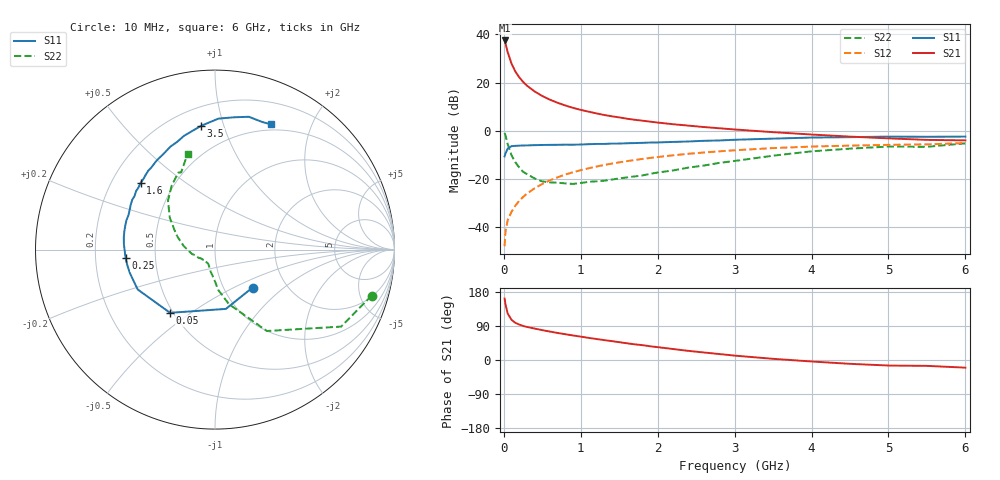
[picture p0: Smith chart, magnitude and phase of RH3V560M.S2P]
! SIEMENS Small Signal Semiconductors
! BFR106
! Si NPN RF Bipolar Junction Transistor in SOT23
! VCE = 3.5 V  IC = 60 mA
! Common Emitter S-Parameters:  August  1996
# GHz  S  MA  R  50
!  f  S11  S21  S12  S22
! GHz  MAG  ANG  MAG  ANG  MAG  ANG  MAG  ANG
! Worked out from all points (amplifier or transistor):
!   36 points, 10 MHz to 6 GHz, reference 50 ohm
!   highest |S21| = 37.5 dB at 10 MHz (marker M1)
!   |S21| within 3 dB of that: start of sweep to 35.55 MHz
!   unconditionally stable (mu >= 1): 220.8 MHz to 2.416 GHz
!   at 250 MHz: K = 1.02, MAG = 22.9 dB, |S12| = -27.4 dB
!   at 1.4 GHz: K = 1.06, MAG = 8.4 dB, |S12| = -13.5 dB
!   at 6 GHz: K = 0.99, MSG = 0.6 dB, |S12| = -5.0 dB
!   S11 on the Smith chart (normalised r, x): 10 MHz: 1.36, -0.63; 50 MHz: 0.48, -0.42; 250 MHz: 0.33, -0.04; 1.6 GHz: 0.32, +0.35; 3.5 GHz: 0.32, +0.84; 6 GHz: 0.43, +1.45
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0.01  0.2975 -45.3  75.12 162.1  0.0041 81.5  0.9091 -16.4
0.02  0.3359 -79.6  66.84 148.0  0.0079 69.0  0.8234 -31.4
0.05  0.4321 -125.4  43 122.6  0.0142 61.3  0.5378 -57.5
0.1  0.4846 -152.7  24.83 105.9  0.0212 63.7  0.3139 -75.6
0.15  0.4918 -164.4  17.03 98.0  0.0284 66.3  0.2245 -85.6
0.2  0.4962 -169.9  12.98 93.6  0.0356 69.0  0.1751 -90.3
0.25  0.5004 -174.8  10.41 89.9  0.0428 70.5  0.1432 -96.1
0.3  0.5021 -178.1  8.719 87.3  0.0503 71.7  0.1277 -100.4
0.4  0.5085 176.6  6.601 83.0  0.0649 72.2  0.1037 -107.7
0.5  0.5126 172.4  5.3 78.8  0.0798 72.4  0.0902 -113.6
0.6  0.5155 168.5  4.442 75.0  0.0952 71.6  0.0861 -118.0
0.7  0.5174 165.0  3.834 71.3  0.1097 70.7  0.0846 -123.4
0.9  0.5188 158.4  3.015 64.7  0.1396 68.4  0.0799 -132.8
1.1  0.5321 151.9  2.515 58.4  0.1686 65.6  0.0882 -140.5
1.3  0.5385 146.4  2.152 52.6  0.1966 62.6  0.0929 -148.3
1.6  0.5566 138.1  1.797 44.1  0.2374 58.1  0.1091 -159.1
2.2  0.593 123.3  1.38 28.9  0.3132 48.7  0.1519 -179.3
2.8  0.636 109.4  1.139 15.7  0.3783 39.1  0.2179 161.8
3.5  0.694 96.4  0.945 3.1  0.4419 28.4  0.3076 144.9
4.5  0.7447 81.8  0.764 -10.1  0.4971 13.9  0.4305 124.1
5.5  0.758 69.8  0.654 -15.5  0.528 4.7  0.4695 113.7
6  0.7642 65.9  0.638 -20.2  0.5601 -2.4  0.5542 106.0
